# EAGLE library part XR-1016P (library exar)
Seventh order switched capacitor FILTER
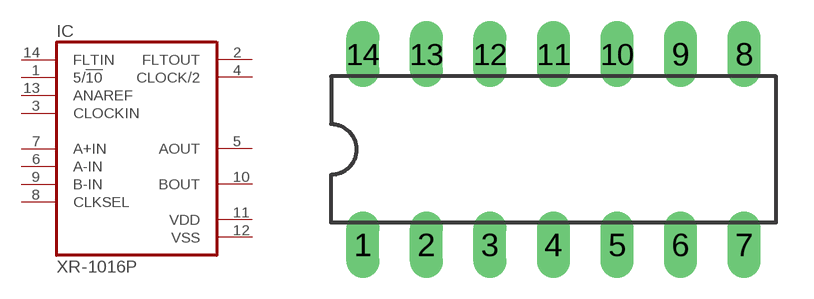
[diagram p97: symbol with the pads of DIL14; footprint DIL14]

Designator prefix IC

## XR-1016P (OC_FARNELL: unknown; OC_NEWARK: unknown)  [DIL14]
1  5/!10  in
2  FLTOUT  out
3  CLOCKIN  in
4  CLOCK/2  out
5  AOUT  out
6  A-IN  in
7  A+IN  in
8  CLKSEL  in
9  B-IN  in
10  BOUT  out
11  VDD  pwr
12  VSS  pwr
13  ANAREF  in
14  FLTIN  in

## Footprint DIL14 (pad centres in mm)
Dual In Line Package
drill 0.813 long: 1 -7.62,-3.81; 2 -5.08,-3.81; 3 -2.54,-3.81; 4 0,-3.81; 5 2.54,-3.81; 6 5.08,-3.81; 7 7.62,-3.81; 8 7.62,3.81; 9 5.08,3.81; 10 2.54,3.81; 11 0,3.81; 12 -2.54,3.81; 13 -5.08,3.81; 14 -7.62,3.81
